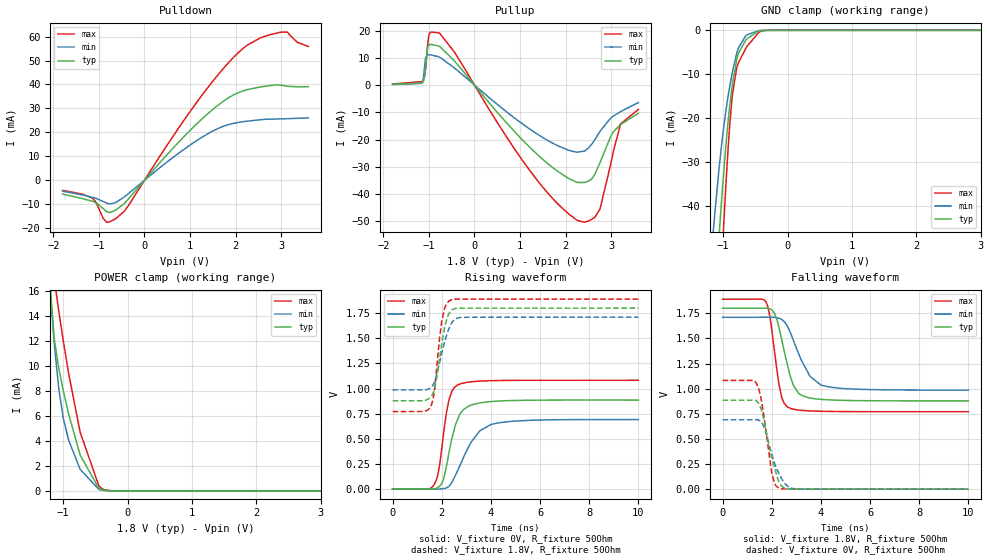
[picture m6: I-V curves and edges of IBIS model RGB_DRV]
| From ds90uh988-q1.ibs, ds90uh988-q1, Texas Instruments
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|  RGB_DRV
[Model]   RGB_DRV
Model_type   Output
Polarity   Non-Inverting
Vmeas = 0.9
Vref = 0.9
Cref = 0.02pF
Rref = 50
|   typ   min   max
C_comp   1.1057pF   1.1578pF   1.2695pF
[Voltage Range]   1.8   1.71   1.89
[Temperature Range]   27   105   -40
[Pullup Reference]   1.8   1.71   1.89
[Pulldown Reference]   -0   -0   0
[Power Clamp Reference]   1.8   1.71   1.89
[GND Clamp Reference]   0   0   0
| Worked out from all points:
|   slope of the pulldown table from 0 to 0.27 V, typ, clamps not added: 45.8 ohm
|   slope of the pullup table from 0 to 0.27 V, typ, clamps not added: 49.3 ohm
|   GND clamp passes 1 mA (typ) near -0.53 V on its own axis
|   falling waveform, V_fixture 1.8V, R_fixture 50Ohm: 20-80 % time 551ps typ, 794ps min, 382ps max; typ from 1.8 V to 0.878 V
|   rising waveform, V_fixture 0V, R_fixture 50Ohm: 20-80 % time 525ps typ, 906ps min, 381ps max; typ from 0 V to 0.885 V
|   rising waveform, V_fixture 1.8V, R_fixture 50Ohm: 20-80 % time 366ps typ, 462ps min, 291ps max; typ from 0.878 V to 1.8 V
|   falling waveform, V_fixture 0V, R_fixture 50Ohm: 20-80 % time 494ps typ, 553ps min, 379ps max; typ from 0.885 V to 0 V
[Pulldown]
|   Voltage   I(typ)   I(min)   I(max)
-1.8V     -5.767mA   -4.594mA   -4.213mA
-1.152V   -8.741mA   -7.097mA   -7.455mA
-833.4mV  -13.09mA   -9.538mA   -17.5mA
-639mV    -12.56mA   -9.365mA   -16.12mA
-369mV    -8.157mA   -5.849mA   -11.04mA
1.143V    23.44mA    16.5mA     32.41mA
2.083V    36.73mA    24.2mA     53.68mA
2.558V    39.02mA    25.31mA    59.58mA
3.006V    39.7mA     25.62mA    61.88mA
3.136V    39.29mA    25.7mA     61.88mA
3.357V    39.04mA    25.86mA    57.63mA
3.6V      39.08mA    26.04mA    55.86mA
[GND Clamp]
|   Voltage   I(typ)   I(min)   I(max)
-1.8V     -225.9mA   -171.2mA   -304.8mA
-1.174V   -71.51mA   -49.3mA    -98.97mA
-1.13V    -61.62mA   -41.95mA   -85.42mA
-1.066V   -47.36mA   -31.81mA   -65.62mA
-1.006V   -35.19mA   -23.82mA   -48.36mA
-952.2mV  -25.38mA   -17.82mA   -33.95mA
-919.8mV  -20.29mA   -14.72mA   -26.26mA
-855mV    -12.2mA    -9.419mA   -14.52mA
-784.8mV  -6.398mA   -5.036mA   -8.357mA
-628.2mV  -1.899mA   -1.008mA   -3.639mA
-342mV    -9.663uA   -7.46uA    -26.57uA
3.6V      0A         0A         0A
[Pullup]
|   Voltage   I(typ)   I(min)   I(max)
-1.8V     268.3uA    190.1uA    379.5uA
-1.136V   966.3uA    1.307mA    1.618mA
-1.076V   6.109mA    9.927mA    5.752mA
-1.033V   13.74mA    10.97mA    13.75mA
-990mV    14.79mA    11.09mA    18.88mA
-779.4mV  14.3mA     10.35mA    19.15mA
1.37V     -25.3mA    -17.88mA   -34.73mA
2.412V    -35.76mA   -24.24mA   -50.32mA
2.758V    -28.5mA    -16.98mA   -45.47mA
2.99V     -18.96mA   -12.16mA   -29.28mA
3.211V    -14.46mA   -9.728mA   -14.23mA
3.6V      -10.38mA   -6.417mA   -8.97mA
[POWER Clamp]
|   Voltage   I(typ)   I(min)   I(max)
-1.8V     141.2mA    82.03mA    283.7mA
-1.222V   17.9mA     17.66mA    20.89mA
-1.136V   12.13mA    11.68mA    16.95mA
-1.071V   9.927mA    8.357mA    14.53mA
-1.066V   9.776mA    8.128mA    14.34mA
-995.4mV  7.987mA    5.766mA    11.95mA
-914.4mV  6.162mA    4.065mA    9.409mA
-736.2mV  2.878mA    1.735mA    4.712mA
-444.6mV  208.3uA    118.9uA    403.4uA
-352.8mV  51.43uA    32.26uA    91.72uA
-190.8mV  2.068uA    1.923uA    3.206uA
3.6V      0A         0A         0A
[Ramp]
R_load = 50
|   typ   min   max
dV/dt_r   0.530931/5.25442e-10   0.414526/9.0603e-10   0.649237/3.80518e-10
dV/dt_f   0.552962/5.50644e-10   0.43454/7.93664e-10   0.671475/3.82261e-10
[Falling Waveform]
V_fixture = 1.8V
V_fixture_min = 1.71V
V_fixture_max = 1.89V
R_fixture = 50Ohm
C_fixture = 0F
|   Time   V(typ)   V(min)   V(max)
0s        1.8V       1.71V      1.89V
1.781ns   1.801V     1.711V     1.857V
1.92ns    1.794V     1.711V     1.726V
2.116ns   1.747V     1.71V      1.365V
2.408ns   1.486V     1.688V     913.5mV
2.797ns   1.091V     1.535V     800.4mV
3.094ns   954.1mV    1.349V     787.6mV
3.557ns   907.5mV    1.123V     778.6mV
3.995ns   894.1mV    1.037V     775.2mV
10ns      878.4mV    985.8mV    770.8mV
[Rising Waveform]
V_fixture = 0V
V_fixture_min = 0V
V_fixture_max = 0V
R_fixture = 50Ohm
C_fixture = 0F
|   Time   V(typ)   V(min)   V(max)
0s        83.74uV    84.63uV    68.95uV
1.443ns   -1.117mV   -579.4uV   -376.7uV
1.696ns   1.655mV    -936.8uV   46.67mV
1.838ns   13.88mV    -598.7uV   136mV
2.05ns    83.56mV    3.08mV     501.3mV
2.297ns   363.1mV    28.06mV    889.2mV
2.633ns   683.1mV    174.9mV    1.034V
3.196ns   834.7mV    467.1mV    1.067V
3.995ns   869.9mV    641mV      1.078V
10ns      885mV      691mV      1.082V
[Rising Waveform]
V_fixture = 1.8V
V_fixture_min = 1.71V
V_fixture_max = 1.89V
R_fixture = 50Ohm
C_fixture = 0F
|   Time   V(typ)   V(min)   V(max)
0s        878.4mV    985.8mV    770.8mV
1.245ns   878.9mV    986.3mV    771.1mV
1.538ns   912mV      1.006V     815.7mV
1.696ns   989.8mV    1.061V     972.7mV
2ns       1.441V     1.35V      1.669V
2.116ns   1.604V     1.46V      1.798V
2.212ns   1.697V     1.538V     1.846V
2.408ns   1.781V     1.654V     1.885V
2.925ns   1.8V       1.708V     1.889V
10ns      1.8V       1.71V      1.89V
[Falling Waveform]
|Gnd
V_fixture = 0V
V_fixture_min = 0V
V_fixture_max = 0V
R_fixture = 50Ohm
C_fixture = 0F
|   Time   V(typ)   V(min)   V(max)
0s        884.9mV    691mV      1.082V
1.384ns   877.3mV    690.8mV    1.049V
1.584ns   784.6mV    663.5mV    876.3mV
1.752ns   604.6mV    571.4mV    604.2mV
2ns       321.2mV    347.4mV    165.4mV
2.116ns   213.9mV    258.7mV    55.62mV
2.297ns   71.32mV    152.9mV    9.911mV
2.622ns   4.534mV    34.23mV    1.303mV
2.925ns   745.7uV    4.625mV    1.146mV
10ns      82.69uV    85.65uV    76.45uV
